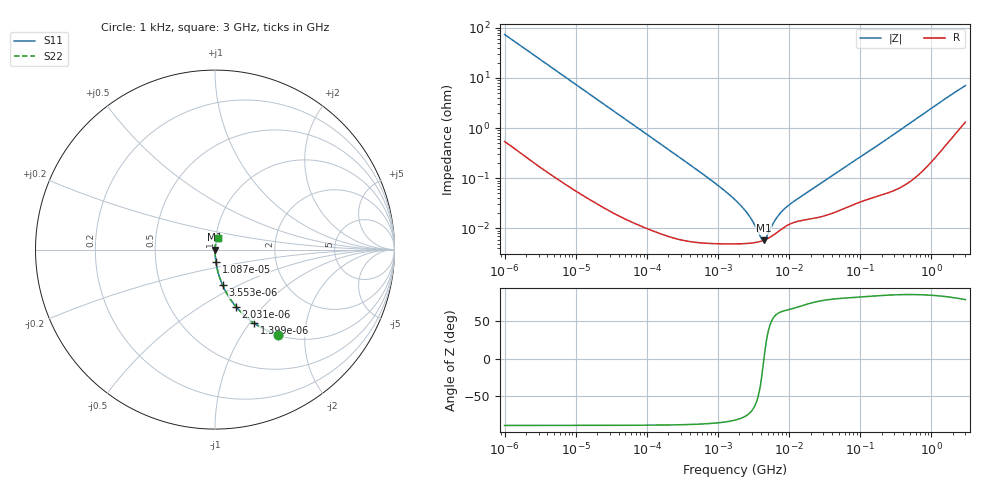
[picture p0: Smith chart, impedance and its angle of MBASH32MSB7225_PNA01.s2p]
! MBASH32MSB7225_PNA01  S-PARAMETER MODEL  ( Standard Model )
! Model Generated by TAIYO YUDEN Corporation (http://www.ty-top.com)
! Version 1.0
! TAIYO YUDEN Control No. 220601
! Copyright(c) 2015 TAIYO YUDEN CO.,LTD. All Rights Reserved.
! Product Description (link to TY-COMPAS)
! https://ds.yuden.co.jp/TYCOMPAS/or/detail?pn=MBASH32MSB7225KPNA01&u=M
! Products Name : Multilayer Ceramic Capacitors
! Characteristics :
!  Capacitance : 2.2 [uF] , Rated Voltage : 100 [V] , TCC : X7R
!  Case Size : 3.2 x 2.5 / 0.126 x 0.098 [mm/inch] , Thickness : 2.5 / 0.098 [mm/inch]
!  (Conditions: Temperature = 25 [degC] , DC Bias Voltage = 0 [V])
! External Node Assignments :
!  1  o---| |---o  2
! GND o---------o GND
! Frequency Range : 1kHz  -  3GHz  [ 401 STEP ]
# MHZ S RI R 50
! Freq[MHz].  S11 Real  S11 Imag  S21 Real  S21 Imag  S12 Real  S12 Imag  S22 Real  S22 Imag
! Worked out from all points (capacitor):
!   401 points, 1 kHz to 3 GHz, reference 50 ohm
!   read as one part in series: C = 2.17 uF near 1.077 kHz
!   lowest |Z| = 5.81 mohm at 4.399 MHz (marker M1)
!   series resonance near 4.423 MHz, so ESL is about 600 pH
!   S11 on the Smith chart (normalised r, x): 1 kHz: 1.01, -1.47; 1.399 kHz: 1.01, -1.05; 2.031 kHz: 1.01, -0.72; 3.553 kHz: 1.00, -0.42; 10.87 kHz: 1.00, -0.14; 3 GHz: 1.03, +0.14
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0.001  0.3507 -0.4735  0.6493 0.4735  0.6493 0.4735  0.3507 -0.4735
0.001399  0.2178 -0.4091  0.7822 0.4091  0.7822 0.4091  0.2178 -0.4091
0.002031  0.1178 -0.3188  0.8822 0.3188  0.8822 0.3188  0.1178 -0.3188
0.003553  0.0426 -0.1985  0.9574 0.1985  0.9574 0.1985  0.0426 -0.1985
0.005988  0.0159 -0.1214  0.9841 0.1214  0.9841 0.1214  0.0159 -0.1214
0.010873  0.00513 -0.0678  0.9949 0.0678  0.9949 0.0678  0.00513 -0.0678
0.01216  0.00417 -0.0607  0.9958 0.0607  0.9958 0.0607  0.00417 -0.0607
0.033275  0.000705 -0.0224  0.9993 0.0224  0.9993 0.0224  0.000705 -0.0224
0.147855  0.000106 -0.00507  0.9999 0.00507  0.9999 0.00507  0.000106 -0.00507
0.791611  5.09e-05 -0.000922  0.9999 0.000922  0.9999 0.000922  5.09e-05 -0.000922
1.732051  4.93e-05 -0.00037  1 0.00037  1 0.00037  4.93e-05 -0.00037
2.422679  4.99e-05 -0.00022  1 0.00022  1 0.00022  4.99e-05 -0.00022
3.517417  5.3e-05 -7.98e-05  0.9999 7.98e-05  0.9999 7.98e-05  5.3e-05 -7.98e-05
4.399271  5.8e-05 -1.85e-06  0.9999 1.85e-06  0.9999 1.85e-06  5.8e-05 -1.85e-06
5.30084  6.59e-05 6.23e-05  0.9999 -6.23e-05  0.9999 -6.23e-05  6.59e-05 6.23e-05
5.711239  7.03e-05 8.78e-05  0.9999 -8.78e-05  0.9999 -8.78e-05  7.03e-05 8.78e-05
7.143107  8.85e-05 0.000163  0.9999 -0.000163  0.9999 -0.000163  8.85e-05 0.000163
8.933959  0.00011 0.000234  0.9999 -0.000234  0.9999 -0.000234  0.00011 0.000234
21.06097  0.000157 0.000589  0.9998 -0.000589  0.9998 -0.000589  0.000157 0.000589
256.0921  0.000564 0.00648  0.9994 -0.00648  0.9994 -0.00648  0.000564 0.00648
1533.384  0.00563 0.0371  0.9944 -0.0371  0.9944 -0.0371  0.00563 0.0371
3000  0.0175 0.0669  0.9825 -0.0669  0.9825 -0.0669  0.0175 0.0669
